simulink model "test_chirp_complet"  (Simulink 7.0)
settings: Solver=FixedStepDiscrete  StartTime=0.0  StopTime=50  FixedStep=Ts  RelTol=1e-3

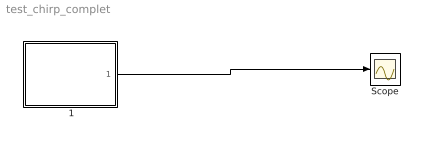
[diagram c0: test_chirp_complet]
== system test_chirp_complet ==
  " 1" : Subsystem  mask{n=2, Fbeg=[60; 90;75], Ffin=[70;100;85], amp=0.1, T0=15, T1=18, Tb=3, T2=3}
      mask prompts: n "level"; Fbeg "Initial frequency sequence (vector Fbeg) [Hz]"; Ffin "Final frequency sequence (vector Ffin) [Hz]"; amp "Amplitude (Amp)"; T0 "Instant of the initial frequency sequence injection 'T0'"; T1 "instant to run a chirp 'T1'"; Tb "Transition time between  Fbeg and Ffin ('Tb') "slope=(Ffin-Fbeg)/Tb""; T2 "Time duration of the final frequency sequence Ffin 'T2'"
  Scope : Scope
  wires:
  " 1"/1(Out2) -> Scope/1

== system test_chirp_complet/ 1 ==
  Constant : Constant  Value=n  OutDataType=sfix(16)  OutScaling=2^0
  Multiport Switch : MultiPortSwitch  Inputs=3  OutDataType=sfix(16)  OutScaling=2^0
  Subsystem : Subsystem
  Subsystem1 : Subsystem
  Subsystem2 : Subsystem
  Out2 : Outport
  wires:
  Constant/1 -> Multiport Switch/1
  Subsystem2/1(Out1) -> Multiport Switch/2
  Subsystem1/1(Out1) -> Multiport Switch/3
  Subsystem/1(Out1) -> Multiport Switch/4
  Multiport Switch/1 -> Out2/1

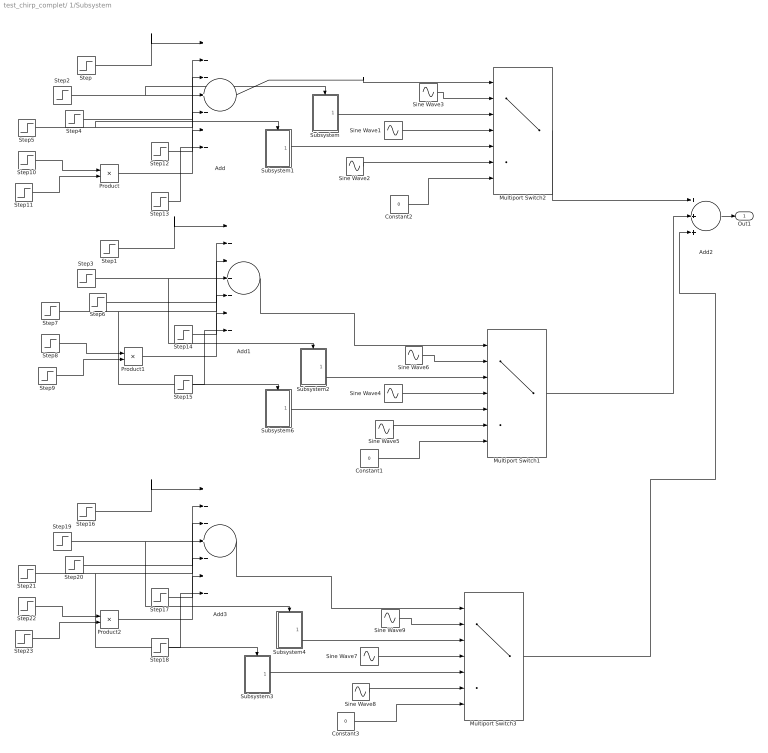
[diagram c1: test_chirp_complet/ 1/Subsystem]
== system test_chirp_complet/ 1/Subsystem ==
  Add : Sum  Inputs=+++++++  OutDataType=sfix(16)  OutScaling=2^-10
  Add1 : Sum  Inputs=+++++++  OutDataType=sfix(16)  OutScaling=2^-10
  Add2 : Sum  Inputs=+++  OutDataType=sfix(16)  OutScaling=2^-10
  Add3 : Sum  Inputs=+++++++  OutDataType=sfix(16)  OutScaling=2^-10
  Constant1 : Constant  Value=0  OutDataType=sfix(16)  OutScaling=2^0
  Constant2 : Constant  Value=0  OutDataType=sfix(16)  OutScaling=2^0
  Constant3 : Constant  Value=0  OutDataType=sfix(16)  OutScaling=2^0
  Multiport Switch1 : MultiPortSwitch  Inputs=6  OutDataType=sfix(16)  OutScaling=2^0
  Multiport Switch2 : MultiPortSwitch  Inputs=6  OutDataType=sfix(16)  OutScaling=2^0
  Multiport Switch3 : MultiPortSwitch  Inputs=6  OutDataType=sfix(16)  OutScaling=2^0
  Product : Product  OutDataType=sfix(16)  OutScaling=2^0
  Product1 : Product  OutDataType=sfix(16)  OutScaling=2^0
  Product2 : Product  OutDataType=sfix(16)  OutScaling=2^0
  Sine Wave1 : Sin  Amplitude=amp  Frequency=Ffin(1)*2*pi  SampleTime=0
  Sine Wave2 : Sin  Amplitude=amp  Frequency=Fbeg(1)*2*pi  SampleTime=0
  Sine Wave3 : Sin  Amplitude=amp  Frequency=Fbeg(1)*2*pi  SampleTime=0
  Sine Wave4 : Sin  Amplitude=amp  Frequency=Ffin(2)*2*pi  SampleTime=0
  Sine Wave5 : Sin  Amplitude=amp  Frequency=Fbeg(2)*2*pi  SampleTime=0
  Sine Wave6 : Sin  Amplitude=amp  Frequency=Fbeg(2)*2*pi  SampleTime=0
  Sine Wave7 : Sin  Amplitude=amp  Frequency=Ffin(3)*2*pi  SampleTime=0
  Sine Wave8 : Sin  Amplitude=amp  Frequency=Fbeg(3)*2*pi  SampleTime=0
  Sine Wave9 : Sin  Amplitude=amp  Frequency=Fbeg(3)*2*pi  SampleTime=0
  Step : Step  Time=T0  SampleTime=0
  Step1 : Step  Time=T0  SampleTime=0
  Step10 : Step  Time=0  After=4  SampleTime=0
  Step11 : Step  Time=T0  Before=1  After=0  SampleTime=0
  Step12 : Step  Time=Tb+T1+T2+Tb  SampleTime=0
  Step13 : Step  Time=Tb+T1+T2+Tb+T2  SampleTime=0
  Step14 : Step  Time=Tb+T1+T2+Tb  SampleTime=0
  Step15 : Step  Time=Tb+T1+T2+Tb+T2  SampleTime=0
  Step16 : Step  Time=T0  SampleTime=0
  Step17 : Step  Time=Tb+T1+T2+Tb  SampleTime=0
  Step18 : Step  Time=Tb+T1+T2+Tb+T2  SampleTime=0
  Step19 : Step  Time=T1  SampleTime=0
  Step2 : Step  Time=T1  SampleTime=0
  Step20 : Step  Time=Tb+T1  SampleTime=0
  Step21 : Step  Time=Tb+T1+T2  SampleTime=0
  Step22 : Step  Time=0  After=4  SampleTime=0
  Step23 : Step  Time=T0  Before=1  After=0  SampleTime=0
  Step3 : Step  Time=T1  SampleTime=0
  Step4 : Step  Time=Tb+T1  SampleTime=0
  Step5 : Step  Time=Tb+T1+T2  SampleTime=0
  Step6 : Step  Time=Tb+T1  SampleTime=0
  Step7 : Step  Time=Tb+T1+T2  SampleTime=0
  Step8 : Step  Time=0  After=4  SampleTime=0
  Step9 : Step  Time=T0  Before=1  After=0  SampleTime=0
  Subsystem : Subsystem
  Subsystem1 : Subsystem
  Subsystem2 : Subsystem
  Subsystem3 : Subsystem
  Subsystem4 : Subsystem
  Subsystem6 : Subsystem
  Out1 : Outport
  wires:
  Add2/1 -> Out1/1
  Subsystem/1(Out1) -> Multiport Switch2/3
  Sine Wave3/1 -> Multiport Switch2/2
  Sine Wave1/1 -> Multiport Switch2/4
  Subsystem1/1(Out1) -> Multiport Switch2/5
  Sine Wave2/1 -> Multiport Switch2/6
  Constant2/1 -> Multiport Switch2/7
  Step/1 -> Add/1
  Step2/1 -> Add/2, Subsystem/Enable
  Step4/1 -> Add/3
  Step5/1 -> Add/4, Subsystem1/Enable
  Step10/1 -> Product/1
  Step11/1 -> Product/2
  Add/1 -> Multiport Switch2/1
  Step12/1 -> Add/5
  Product/1 -> Add/6
  Multiport Switch2/1 -> Add2/1
  Step13/1 -> Add/7
  Subsystem2/1(Out1) -> Multiport Switch1/3
  Sine Wave6/1 -> Multiport Switch1/2
  Sine Wave4/1 -> Multiport Switch1/4
  Subsystem6/1(Out1) -> Multiport Switch1/5
  Sine Wave5/1 -> Multiport Switch1/6
  Constant1/1 -> Multiport Switch1/7
  Step1/1 -> Add1/1
  Step3/1 -> Add1/2, Subsystem2/Enable
  Step6/1 -> Add1/3
  Step7/1 -> Add1/4, Subsystem6/Enable
  Step8/1 -> Product1/1
  Step9/1 -> Product1/2
  Add1/1 -> Multiport Switch1/1
  Step14/1 -> Add1/5
  Product1/1 -> Add1/6
  Multiport Switch1/1 -> Add2/2
  Step15/1 -> Add1/7
  Subsystem4/1(Out1) -> Multiport Switch3/3
  Sine Wave9/1 -> Multiport Switch3/2
  Sine Wave7/1 -> Multiport Switch3/4
  Subsystem3/1(Out1) -> Multiport Switch3/5
  Sine Wave8/1 -> Multiport Switch3/6
  Constant3/1 -> Multiport Switch3/7
  Step16/1 -> Add3/1
  Step19/1 -> Add3/2, Subsystem4/Enable
  Step20/1 -> Add3/3
  Step21/1 -> Add3/4, Subsystem3/Enable
  Step22/1 -> Product2/1
  Step23/1 -> Product2/2
  Add3/1 -> Multiport Switch3/1
  Step17/1 -> Add3/5
  Product2/1 -> Add3/6
  Multiport Switch3/1 -> Add2/3
  Step18/1 -> Add3/7

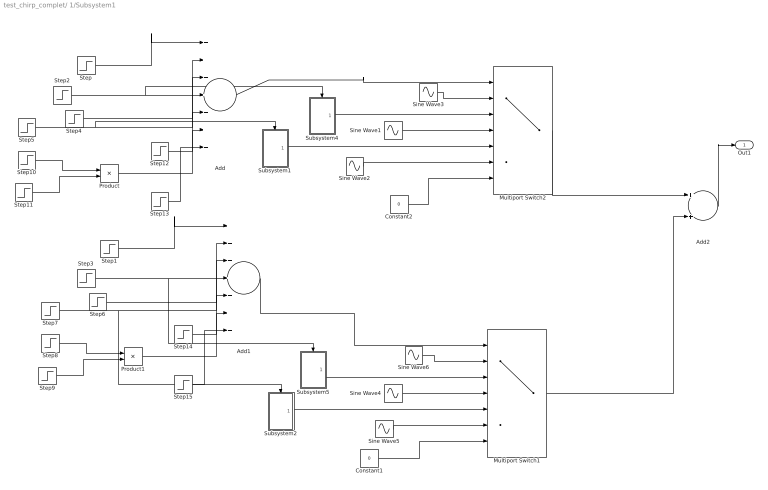
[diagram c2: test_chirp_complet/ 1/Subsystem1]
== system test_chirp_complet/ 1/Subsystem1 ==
  Add : Sum  Inputs=+++++++  OutDataType=sfix(16)  OutScaling=2^-10
  Add1 : Sum  Inputs=+++++++  OutDataType=sfix(16)  OutScaling=2^-10
  Add2 : Sum  OutDataType=sfix(16)  OutScaling=2^-10
  Constant1 : Constant  Value=0  OutDataType=sfix(16)  OutScaling=2^0
  Constant2 : Constant  Value=0  OutDataType=sfix(16)  OutScaling=2^0
  Multiport Switch1 : MultiPortSwitch  Inputs=6  OutDataType=sfix(16)  OutScaling=2^0
  Multiport Switch2 : MultiPortSwitch  Inputs=6  OutDataType=sfix(16)  OutScaling=2^0
  Product : Product  OutDataType=sfix(16)  OutScaling=2^0
  Product1 : Product  OutDataType=sfix(16)  OutScaling=2^0
  Sine Wave1 : Sin  Amplitude=amp  Frequency=Ffin(1)*2*pi  SampleTime=0
  Sine Wave2 : Sin  Amplitude=amp  Frequency=Fbeg(1)*2*pi  SampleTime=0
  Sine Wave3 : Sin  Amplitude=amp  Frequency=Fbeg(1)*2*pi  SampleTime=0
  Sine Wave4 : Sin  Amplitude=amp  Frequency=Ffin(2)*2*pi  SampleTime=0
  Sine Wave5 : Sin  Amplitude=amp  Frequency=Fbeg(2)*2*pi  SampleTime=0
  Sine Wave6 : Sin  Amplitude=amp  Frequency=Fbeg(2)*2*pi  SampleTime=0
  Step : Step  Time=T0  SampleTime=0
  Step1 : Step  Time=T0  SampleTime=0
  Step10 : Step  Time=0  After=4  SampleTime=0
  Step11 : Step  Time=T0  Before=1  After=0  SampleTime=0
  Step12 : Step  Time=Tb+T1+T2+Tb  SampleTime=0
  Step13 : Step  Time=Tb+T1+T2+Tb+T2  SampleTime=0
  Step14 : Step  Time=Tb+T1+T2+Tb  SampleTime=0
  Step15 : Step  Time=Tb+T1+T2+Tb+T2  SampleTime=0
  Step2 : Step  Time=T1  SampleTime=0
  Step3 : Step  Time=T1  SampleTime=0
  Step4 : Step  Time=Tb+T1  SampleTime=0
  Step5 : Step  Time=Tb+T1+T2  SampleTime=0
  Step6 : Step  Time=Tb+T1  SampleTime=0
  Step7 : Step  Time=Tb+T1+T2  SampleTime=0
  Step8 : Step  Time=0  After=4  SampleTime=0
  Step9 : Step  Time=T0  Before=1  After=0  SampleTime=0
  Subsystem1 : Subsystem
  Subsystem2 : Subsystem
  Subsystem4 : Subsystem
  Subsystem5 : Subsystem
  Out1 : Outport
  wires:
  Add2/1 -> Out1/1
  Subsystem4/1(Out1) -> Multiport Switch2/3
  Sine Wave3/1 -> Multiport Switch2/2
  Sine Wave1/1 -> Multiport Switch2/4
  Subsystem1/1(Out1) -> Multiport Switch2/5
  Sine Wave2/1 -> Multiport Switch2/6
  Constant2/1 -> Multiport Switch2/7
  Step/1 -> Add/1
  Step2/1 -> Add/2, Subsystem4/Enable
  Step4/1 -> Add/3
  Step5/1 -> Add/4, Subsystem1/Enable
  Step10/1 -> Product/1
  Step11/1 -> Product/2
  Add/1 -> Multiport Switch2/1
  Step12/1 -> Add/5
  Product/1 -> Add/6
  Multiport Switch2/1 -> Add2/1
  Step13/1 -> Add/7
  Subsystem5/1(Out1) -> Multiport Switch1/3
  Sine Wave6/1 -> Multiport Switch1/2
  Sine Wave4/1 -> Multiport Switch1/4
  Subsystem2/1(Out1) -> Multiport Switch1/5
  Sine Wave5/1 -> Multiport Switch1/6
  Constant1/1 -> Multiport Switch1/7
  Step1/1 -> Add1/1
  Step3/1 -> Add1/2, Subsystem5/Enable
  Step6/1 -> Add1/3
  Step7/1 -> Add1/4, Subsystem2/Enable
  Step8/1 -> Product1/1
  Step9/1 -> Product1/2
  Add1/1 -> Multiport Switch1/1
  Step14/1 -> Add1/5
  Product1/1 -> Add1/6
  Multiport Switch1/1 -> Add2/2
  Step15/1 -> Add1/7

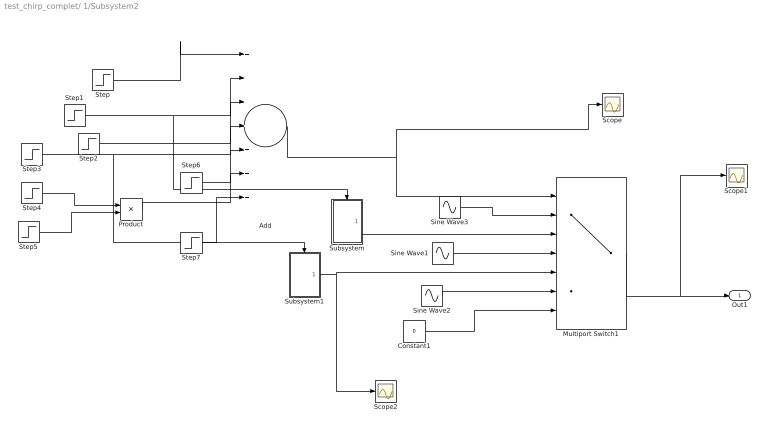
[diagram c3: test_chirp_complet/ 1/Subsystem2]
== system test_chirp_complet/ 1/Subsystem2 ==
  Add : Sum  Inputs=+++++++  OutDataType=sfix(16)  OutScaling=2^-10
  Constant1 : Constant  Value=0  OutDataType=sfix(16)  OutScaling=2^0
  Multiport Switch1 : MultiPortSwitch  Inputs=6  OutDataType=sfix(16)  OutScaling=2^0
  Product : Product  OutDataType=sfix(16)  OutScaling=2^0
  Scope : Scope
  Scope1 : Scope
  Scope2 : Scope
  Sine Wave1 : Sin  Amplitude=amp  Frequency=Ffin(1)*2*pi  SampleTime=0
  Sine Wave2 : Sin  Amplitude=amp  Frequency=Fbeg(1)*2*pi  SampleTime=0
  Sine Wave3 : Sin  Amplitude=amp  Frequency=Fbeg(1)*2*pi  SampleTime=0
  Step : Step  Time=T0  SampleTime=0
  Step1 : Step  Time=T1  SampleTime=0
  Step2 : Step  Time=Tb+T1  SampleTime=0
  Step3 : Step  Time=Tb+T1+T2  SampleTime=0
  Step4 : Step  Time=0  After=4  SampleTime=0
  Step5 : Step  Time=T0  Before=1  After=0  SampleTime=0
  Step6 : Step  Time=Tb+T1+T2+Tb  SampleTime=0
  Step7 : Step  Time=Tb+T1+T2+Tb+T2  SampleTime=0
  Subsystem : Subsystem
  Subsystem1 : Subsystem
  Out1 : Outport
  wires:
  Subsystem/1(Out1) -> Multiport Switch1/3
  Sine Wave3/1 -> Multiport Switch1/2
  Sine Wave1/1 -> Multiport Switch1/4
  Subsystem1/1(Out1) -> Multiport Switch1/5, Scope2/1
  Sine Wave2/1 -> Multiport Switch1/6
  Constant1/1 -> Multiport Switch1/7
  Step/1 -> Add/1
  Step1/1 -> Add/2, Subsystem/Enable
  Step2/1 -> Add/3
  Step3/1 -> Add/4, Subsystem1/Enable
  Step4/1 -> Product/1
  Step5/1 -> Product/2
  Add/1 -> Multiport Switch1/1, Scope/1
  Step6/1 -> Add/5
  Product/1 -> Add/6
  Multiport Switch1/1 -> Out1/1, Scope1/1
  Step7/1 -> Add/7

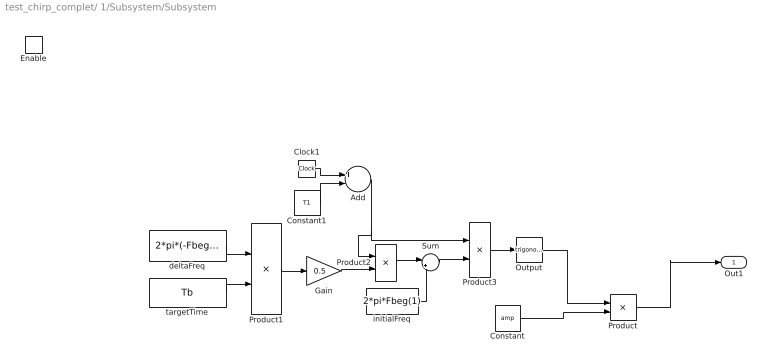
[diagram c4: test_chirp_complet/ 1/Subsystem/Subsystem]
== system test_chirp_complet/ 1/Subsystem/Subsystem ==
  Enable : EnablePort
  Add : Sum  Inputs=+-  OutDataType=sfix(16)  OutScaling=2^-10
  Clock1 : Clock
  Constant : Constant  Value=amp  OutDataType=sfix(16)  OutScaling=2^0
  Constant1 : Constant  Value=T1  OutDataType=sfix(16)  OutScaling=2^0
  Gain : Gain  Gain=0.5  ParameterDataType=sfix(16)  ParameterScaling=2^0  OutDataType=sfix(16)  OutScaling=2^0
  Output : Trigonometry
  Product : Product  OutDataType=sfix(16)  OutScaling=2^0
  Product1 : Product  Inputs=*/  OutDataType=sfix(16)  OutScaling=2^0
  Product2 : Product  OutDataType=sfix(16)  OutScaling=2^0
  Product3 : Product  OutDataType=sfix(16)  OutScaling=2^0
  Sum : Sum  Inputs=|++  OutDataType=sfix(16)  OutScaling=2^0
  deltaFreq : Constant  Value=2*pi*(-Fbeg(1)+Ffin(1))  OutDataType=sfix(16)  OutScaling=2^0
  initialFreq : Constant  Value=2*pi*Fbeg(1)  OutDataType=sfix(16)  OutScaling=2^0
  targetTime : Constant  Value=Tb  OutDataType=sfix(16)  OutScaling=2^0
  Out1 : Outport
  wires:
  Constant/1 -> Product/2
  Output/1 -> Product/1
  Product/1 -> Out1/1
  Product3/1 -> Output/1
  Sum/1 -> Product3/2
  initialFreq/1 -> Sum/2
  Product2/1 -> Sum/1
  Gain/1 -> Product2/2
  Product1/1 -> Gain/1
  targetTime/1 -> Product1/2
  deltaFreq/1 -> Product1/1
  Clock1/1 -> Add/1
  Constant1/1 -> Add/2
  Add/1 -> Product2/1, Product3/1

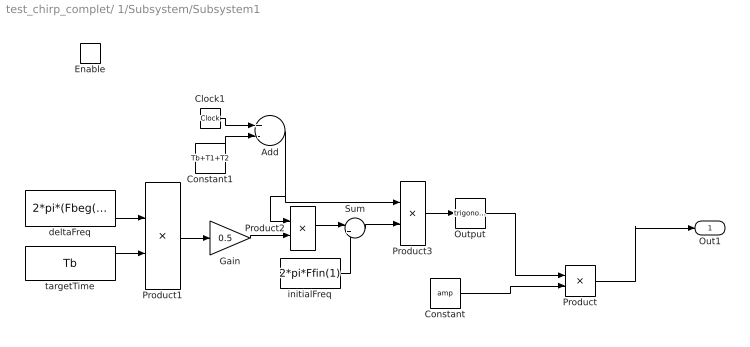
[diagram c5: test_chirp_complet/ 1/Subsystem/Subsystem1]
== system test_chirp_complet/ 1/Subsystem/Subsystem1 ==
  Enable : EnablePort
  Add : Sum  Inputs=+-  OutDataType=sfix(16)  OutScaling=2^-10
  Clock1 : Clock
  Constant : Constant  Value=amp  OutDataType=sfix(16)  OutScaling=2^0
  Constant1 : Constant  Value=Tb+T1+T2  OutDataType=sfix(16)  OutScaling=2^0
  Gain : Gain  Gain=0.5  ParameterDataType=sfix(16)  ParameterScaling=2^0  OutDataType=sfix(16)  OutScaling=2^0
  Output : Trigonometry
  Product : Product  OutDataType=sfix(16)  OutScaling=2^0
  Product1 : Product  Inputs=*/  OutDataType=sfix(16)  OutScaling=2^0
  Product2 : Product  OutDataType=sfix(16)  OutScaling=2^0
  Product3 : Product  OutDataType=sfix(16)  OutScaling=2^0
  Sum : Sum  Inputs=|++  OutDataType=sfix(16)  OutScaling=2^0
  deltaFreq : Constant  Value=2*pi*(Fbeg(1)-Ffin(1))  OutDataType=sfix(16)  OutScaling=2^0
  initialFreq : Constant  Value=2*pi*Ffin(1)  OutDataType=sfix(16)  OutScaling=2^0
  targetTime : Constant  Value=Tb  OutDataType=sfix(16)  OutScaling=2^0
  Out1 : Outport
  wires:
  Add/1 -> Product3/1, Product2/1
  Constant1/1 -> Add/2
  Clock1/1 -> Add/1
  deltaFreq/1 -> Product1/1
  targetTime/1 -> Product1/2
  Product1/1 -> Gain/1
  Gain/1 -> Product2/2
  Product2/1 -> Sum/1
  initialFreq/1 -> Sum/2
  Sum/1 -> Product3/2
  Product3/1 -> Output/1
  Product/1 -> Out1/1
  Output/1 -> Product/1
  Constant/1 -> Product/2

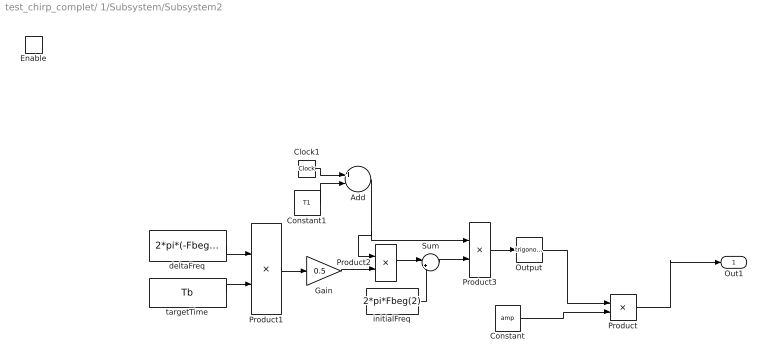
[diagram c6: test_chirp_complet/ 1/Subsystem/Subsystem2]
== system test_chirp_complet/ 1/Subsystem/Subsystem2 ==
  Enable : EnablePort
  Add : Sum  Inputs=+-  OutDataType=sfix(16)  OutScaling=2^-10
  Clock1 : Clock
  Constant : Constant  Value=amp  OutDataType=sfix(16)  OutScaling=2^0
  Constant1 : Constant  Value=T1  OutDataType=sfix(16)  OutScaling=2^0
  Gain : Gain  Gain=0.5  ParameterDataType=sfix(16)  ParameterScaling=2^0  OutDataType=sfix(16)  OutScaling=2^0
  Output : Trigonometry
  Product : Product  OutDataType=sfix(16)  OutScaling=2^0
  Product1 : Product  Inputs=*/  OutDataType=sfix(16)  OutScaling=2^0
  Product2 : Product  OutDataType=sfix(16)  OutScaling=2^0
  Product3 : Product  OutDataType=sfix(16)  OutScaling=2^0
  Sum : Sum  Inputs=|++  OutDataType=sfix(16)  OutScaling=2^0
  deltaFreq : Constant  Value=2*pi*(-Fbeg(2)+Ffin(2))  OutDataType=sfix(16)  OutScaling=2^0
  initialFreq : Constant  Value=2*pi*Fbeg(2)  OutDataType=sfix(16)  OutScaling=2^0
  targetTime : Constant  Value=Tb  OutDataType=sfix(16)  OutScaling=2^0
  Out1 : Outport
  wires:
  Add/1 -> Product3/1, Product2/1
  Constant1/1 -> Add/2
  Clock1/1 -> Add/1
  deltaFreq/1 -> Product1/1
  targetTime/1 -> Product1/2
  Product1/1 -> Gain/1
  Gain/1 -> Product2/2
  Product2/1 -> Sum/1
  initialFreq/1 -> Sum/2
  Sum/1 -> Product3/2
  Product3/1 -> Output/1
  Product/1 -> Out1/1
  Output/1 -> Product/1
  Constant/1 -> Product/2

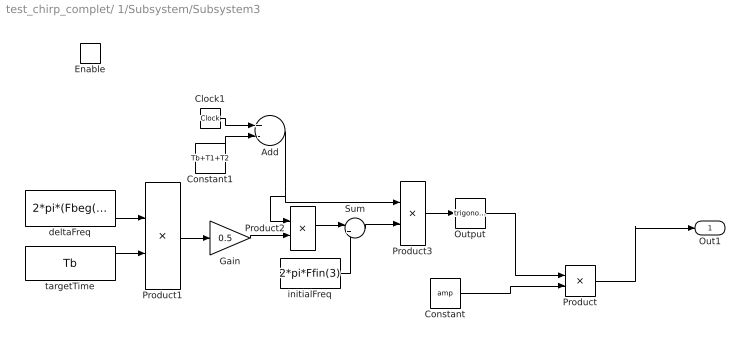
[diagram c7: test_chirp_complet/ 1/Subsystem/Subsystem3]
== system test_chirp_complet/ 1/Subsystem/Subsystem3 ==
  Enable : EnablePort
  Add : Sum  Inputs=+-  OutDataType=sfix(16)  OutScaling=2^-10
  Clock1 : Clock
  Constant : Constant  Value=amp  OutDataType=sfix(16)  OutScaling=2^0
  Constant1 : Constant  Value=Tb+T1+T2  OutDataType=sfix(16)  OutScaling=2^0
  Gain : Gain  Gain=0.5  ParameterDataType=sfix(16)  ParameterScaling=2^0  OutDataType=sfix(16)  OutScaling=2^0
  Output : Trigonometry
  Product : Product  OutDataType=sfix(16)  OutScaling=2^0
  Product1 : Product  Inputs=*/  OutDataType=sfix(16)  OutScaling=2^0
  Product2 : Product  OutDataType=sfix(16)  OutScaling=2^0
  Product3 : Product  OutDataType=sfix(16)  OutScaling=2^0
  Sum : Sum  Inputs=|++  OutDataType=sfix(16)  OutScaling=2^0
  deltaFreq : Constant  Value=2*pi*(Fbeg(3)-Ffin(3))  OutDataType=sfix(16)  OutScaling=2^0
  initialFreq : Constant  Value=2*pi*Ffin(3)  OutDataType=sfix(16)  OutScaling=2^0
  targetTime : Constant  Value=Tb  OutDataType=sfix(16)  OutScaling=2^0
  Out1 : Outport
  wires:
  Add/1 -> Product3/1, Product2/1
  Constant1/1 -> Add/2
  Clock1/1 -> Add/1
  deltaFreq/1 -> Product1/1
  targetTime/1 -> Product1/2
  Product1/1 -> Gain/1
  Gain/1 -> Product2/2
  Product2/1 -> Sum/1
  initialFreq/1 -> Sum/2
  Sum/1 -> Product3/2
  Product3/1 -> Output/1
  Product/1 -> Out1/1
  Output/1 -> Product/1
  Constant/1 -> Product/2

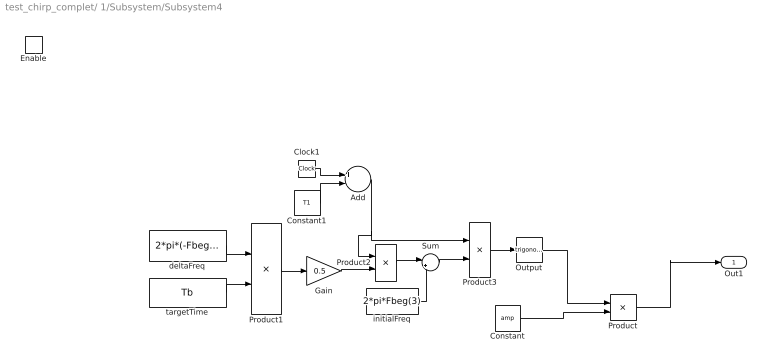
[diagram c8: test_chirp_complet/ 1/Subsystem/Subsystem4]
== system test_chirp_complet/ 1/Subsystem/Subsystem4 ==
  Enable : EnablePort
  Add : Sum  Inputs=+-  OutDataType=sfix(16)  OutScaling=2^-10
  Clock1 : Clock
  Constant : Constant  Value=amp  OutDataType=sfix(16)  OutScaling=2^0
  Constant1 : Constant  Value=T1  OutDataType=sfix(16)  OutScaling=2^0
  Gain : Gain  Gain=0.5  ParameterDataType=sfix(16)  ParameterScaling=2^0  OutDataType=sfix(16)  OutScaling=2^0
  Output : Trigonometry
  Product : Product  OutDataType=sfix(16)  OutScaling=2^0
  Product1 : Product  Inputs=*/  OutDataType=sfix(16)  OutScaling=2^0
  Product2 : Product  OutDataType=sfix(16)  OutScaling=2^0
  Product3 : Product  OutDataType=sfix(16)  OutScaling=2^0
  Sum : Sum  Inputs=|++  OutDataType=sfix(16)  OutScaling=2^0
  deltaFreq : Constant  Value=2*pi*(-Fbeg(3)+Ffin(3))  OutDataType=sfix(16)  OutScaling=2^0
  initialFreq : Constant  Value=2*pi*Fbeg(3)  OutDataType=sfix(16)  OutScaling=2^0
  targetTime : Constant  Value=Tb  OutDataType=sfix(16)  OutScaling=2^0
  Out1 : Outport
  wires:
  Constant/1 -> Product/2
  Output/1 -> Product/1
  Product/1 -> Out1/1
  Product3/1 -> Output/1
  Sum/1 -> Product3/2
  initialFreq/1 -> Sum/2
  Product2/1 -> Sum/1
  Gain/1 -> Product2/2
  Product1/1 -> Gain/1
  targetTime/1 -> Product1/2
  deltaFreq/1 -> Product1/1
  Clock1/1 -> Add/1
  Constant1/1 -> Add/2
  Add/1 -> Product2/1, Product3/1

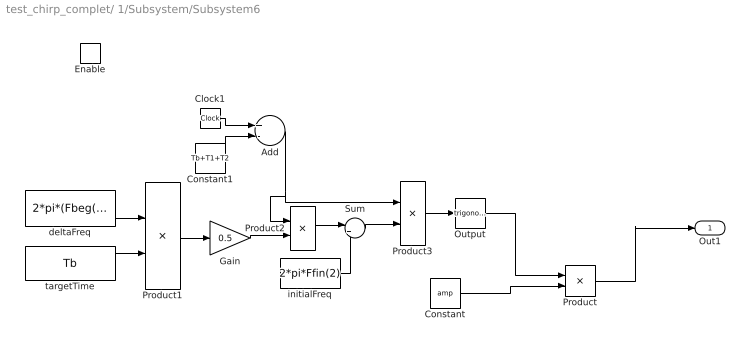
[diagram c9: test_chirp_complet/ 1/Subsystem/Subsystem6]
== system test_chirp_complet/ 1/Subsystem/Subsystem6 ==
  Enable : EnablePort
  Add : Sum  Inputs=+-  OutDataType=sfix(16)  OutScaling=2^-10
  Clock1 : Clock
  Constant : Constant  Value=amp  OutDataType=sfix(16)  OutScaling=2^0
  Constant1 : Constant  Value=Tb+T1+T2  OutDataType=sfix(16)  OutScaling=2^0
  Gain : Gain  Gain=0.5  ParameterDataType=sfix(16)  ParameterScaling=2^0  OutDataType=sfix(16)  OutScaling=2^0
  Output : Trigonometry
  Product : Product  OutDataType=sfix(16)  OutScaling=2^0
  Product1 : Product  Inputs=*/  OutDataType=sfix(16)  OutScaling=2^0
  Product2 : Product  OutDataType=sfix(16)  OutScaling=2^0
  Product3 : Product  OutDataType=sfix(16)  OutScaling=2^0
  Sum : Sum  Inputs=|++  OutDataType=sfix(16)  OutScaling=2^0
  deltaFreq : Constant  Value=2*pi*(Fbeg(2)-Ffin(2))  OutDataType=sfix(16)  OutScaling=2^0
  initialFreq : Constant  Value=2*pi*Ffin(2)  OutDataType=sfix(16)  OutScaling=2^0
  targetTime : Constant  Value=Tb  OutDataType=sfix(16)  OutScaling=2^0
  Out1 : Outport
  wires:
  Constant/1 -> Product/2
  Output/1 -> Product/1
  Product/1 -> Out1/1
  Product3/1 -> Output/1
  Sum/1 -> Product3/2
  initialFreq/1 -> Sum/2
  Product2/1 -> Sum/1
  Gain/1 -> Product2/2
  Product1/1 -> Gain/1
  targetTime/1 -> Product1/2
  deltaFreq/1 -> Product1/1
  Clock1/1 -> Add/1
  Constant1/1 -> Add/2
  Add/1 -> Product2/1, Product3/1

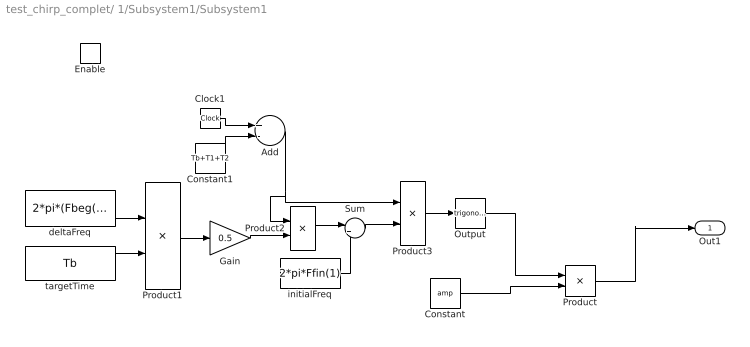
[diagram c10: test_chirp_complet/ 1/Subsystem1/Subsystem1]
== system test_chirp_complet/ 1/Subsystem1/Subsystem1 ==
  Enable : EnablePort
  Add : Sum  Inputs=+-  OutDataType=sfix(16)  OutScaling=2^-10
  Clock1 : Clock
  Constant : Constant  Value=amp  OutDataType=sfix(16)  OutScaling=2^0
  Constant1 : Constant  Value=Tb+T1+T2  OutDataType=sfix(16)  OutScaling=2^0
  Gain : Gain  Gain=0.5  ParameterDataType=sfix(16)  ParameterScaling=2^0  OutDataType=sfix(16)  OutScaling=2^0
  Output : Trigonometry
  Product : Product  OutDataType=sfix(16)  OutScaling=2^0
  Product1 : Product  Inputs=*/  OutDataType=sfix(16)  OutScaling=2^0
  Product2 : Product  OutDataType=sfix(16)  OutScaling=2^0
  Product3 : Product  OutDataType=sfix(16)  OutScaling=2^0
  Sum : Sum  Inputs=|++  OutDataType=sfix(16)  OutScaling=2^0
  deltaFreq : Constant  Value=2*pi*(Fbeg(1)-Ffin(1))  OutDataType=sfix(16)  OutScaling=2^0
  initialFreq : Constant  Value=2*pi*Ffin(1)  OutDataType=sfix(16)  OutScaling=2^0
  targetTime : Constant  Value=Tb  OutDataType=sfix(16)  OutScaling=2^0
  Out1 : Outport
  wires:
  Constant/1 -> Product/2
  Output/1 -> Product/1
  Product/1 -> Out1/1
  Product3/1 -> Output/1
  Sum/1 -> Product3/2
  initialFreq/1 -> Sum/2
  Product2/1 -> Sum/1
  Gain/1 -> Product2/2
  Product1/1 -> Gain/1
  targetTime/1 -> Product1/2
  deltaFreq/1 -> Product1/1
  Clock1/1 -> Add/1
  Constant1/1 -> Add/2
  Add/1 -> Product2/1, Product3/1

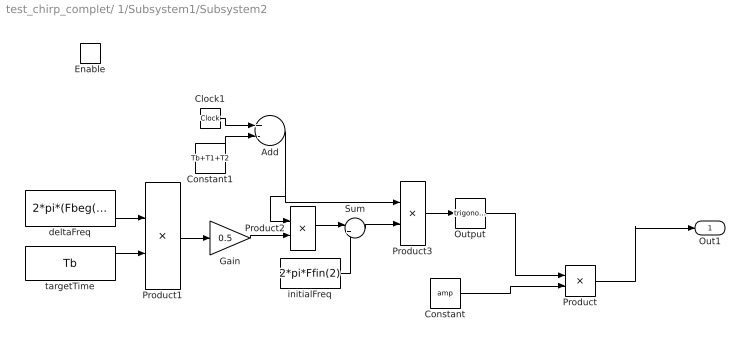
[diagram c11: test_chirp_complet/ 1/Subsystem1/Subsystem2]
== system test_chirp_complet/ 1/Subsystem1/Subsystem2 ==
  Enable : EnablePort
  Add : Sum  Inputs=+-  OutDataType=sfix(16)  OutScaling=2^-10
  Clock1 : Clock
  Constant : Constant  Value=amp  OutDataType=sfix(16)  OutScaling=2^0
  Constant1 : Constant  Value=Tb+T1+T2  OutDataType=sfix(16)  OutScaling=2^0
  Gain : Gain  Gain=0.5  ParameterDataType=sfix(16)  ParameterScaling=2^0  OutDataType=sfix(16)  OutScaling=2^0
  Output : Trigonometry
  Product : Product  OutDataType=sfix(16)  OutScaling=2^0
  Product1 : Product  Inputs=*/  OutDataType=sfix(16)  OutScaling=2^0
  Product2 : Product  OutDataType=sfix(16)  OutScaling=2^0
  Product3 : Product  OutDataType=sfix(16)  OutScaling=2^0
  Sum : Sum  Inputs=|++  OutDataType=sfix(16)  OutScaling=2^0
  deltaFreq : Constant  Value=2*pi*(Fbeg(2)-Ffin(2))  OutDataType=sfix(16)  OutScaling=2^0
  initialFreq : Constant  Value=2*pi*Ffin(2)  OutDataType=sfix(16)  OutScaling=2^0
  targetTime : Constant  Value=Tb  OutDataType=sfix(16)  OutScaling=2^0
  Out1 : Outport
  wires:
  Add/1 -> Product3/1, Product2/1
  Constant1/1 -> Add/2
  Clock1/1 -> Add/1
  deltaFreq/1 -> Product1/1
  targetTime/1 -> Product1/2
  Product1/1 -> Gain/1
  Gain/1 -> Product2/2
  Product2/1 -> Sum/1
  initialFreq/1 -> Sum/2
  Sum/1 -> Product3/2
  Product3/1 -> Output/1
  Product/1 -> Out1/1
  Output/1 -> Product/1
  Constant/1 -> Product/2

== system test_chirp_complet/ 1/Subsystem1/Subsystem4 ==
  Enable : EnablePort
  Add : Sum  Inputs=+-  OutDataType=sfix(16)  OutScaling=2^-10
  Clock1 : Clock
  Constant : Constant  Value=amp  OutDataType=sfix(16)  OutScaling=2^0
  Constant1 : Constant  Value=T1  OutDataType=sfix(16)  OutScaling=2^0
  Gain : Gain  Gain=0.5  ParameterDataType=sfix(16)  ParameterScaling=2^0  OutDataType=sfix(16)  OutScaling=2^0
  Output : Trigonometry
  Product : Product  OutDataType=sfix(16)  OutScaling=2^0
  Product1 : Product  Inputs=*/  OutDataType=sfix(16)  OutScaling=2^0
  Product2 : Product  OutDataType=sfix(16)  OutScaling=2^0
  Product3 : Product  OutDataType=sfix(16)  OutScaling=2^0
  Sum : Sum  Inputs=|++  OutDataType=sfix(16)  OutScaling=2^0
  deltaFreq : Constant  Value=2*pi*(-Fbeg(1)+Ffin(1))  OutDataType=sfix(16)  OutScaling=2^0
  initialFreq : Constant  Value=2*pi*Fbeg(1)  OutDataType=sfix(16)  OutScaling=2^0
  targetTime : Constant  Value=Tb  OutDataType=sfix(16)  OutScaling=2^0
  Out1 : Outport
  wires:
  Constant/1 -> Product/2
  Output/1 -> Product/1
  Product/1 -> Out1/1
  Product3/1 -> Output/1
  Sum/1 -> Product3/2
  initialFreq/1 -> Sum/2
  Product2/1 -> Sum/1
  Gain/1 -> Product2/2
  Product1/1 -> Gain/1
  targetTime/1 -> Product1/2
  deltaFreq/1 -> Product1/1
  Clock1/1 -> Add/1
  Constant1/1 -> Add/2
  Add/1 -> Product2/1, Product3/1

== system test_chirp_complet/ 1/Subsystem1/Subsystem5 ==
  Enable : EnablePort
  Add : Sum  Inputs=+-  OutDataType=sfix(16)  OutScaling=2^-10
  Clock1 : Clock
  Constant : Constant  Value=amp  OutDataType=sfix(16)  OutScaling=2^0
  Constant1 : Constant  Value=T1  OutDataType=sfix(16)  OutScaling=2^0
  Gain : Gain  Gain=0.5  ParameterDataType=sfix(16)  ParameterScaling=2^0  OutDataType=sfix(16)  OutScaling=2^0
  Output : Trigonometry
  Product : Product  OutDataType=sfix(16)  OutScaling=2^0
  Product1 : Product  Inputs=*/  OutDataType=sfix(16)  OutScaling=2^0
  Product2 : Product  OutDataType=sfix(16)  OutScaling=2^0
  Product3 : Product  OutDataType=sfix(16)  OutScaling=2^0
  Sum : Sum  Inputs=|++  OutDataType=sfix(16)  OutScaling=2^0
  deltaFreq : Constant  Value=2*pi*(-Fbeg(2)+Ffin(2))  OutDataType=sfix(16)  OutScaling=2^0
  initialFreq : Constant  Value=2*pi*Fbeg(2)  OutDataType=sfix(16)  OutScaling=2^0
  targetTime : Constant  Value=Tb  OutDataType=sfix(16)  OutScaling=2^0
  Out1 : Outport
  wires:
  Add/1 -> Product3/1, Product2/1
  Constant1/1 -> Add/2
  Clock1/1 -> Add/1
  deltaFreq/1 -> Product1/1
  targetTime/1 -> Product1/2
  Product1/1 -> Gain/1
  Gain/1 -> Product2/2
  Product2/1 -> Sum/1
  initialFreq/1 -> Sum/2
  Sum/1 -> Product3/2
  Product3/1 -> Output/1
  Product/1 -> Out1/1
  Output/1 -> Product/1
  Constant/1 -> Product/2

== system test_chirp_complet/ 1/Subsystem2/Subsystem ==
  Enable : EnablePort
  Add : Sum  Inputs=+-  OutDataType=sfix(16)  OutScaling=2^-10
  Clock1 : Clock
  Constant : Constant  Value=amp  OutDataType=sfix(16)  OutScaling=2^0
  Constant1 : Constant  Value=T1  OutDataType=sfix(16)  OutScaling=2^0
  Gain : Gain  Gain=0.5  ParameterDataType=sfix(16)  ParameterScaling=2^0  OutDataType=sfix(16)  OutScaling=2^0
  Output : Trigonometry
  Product : Product  OutDataType=sfix(16)  OutScaling=2^0
  Product1 : Product  Inputs=*/  OutDataType=sfix(16)  OutScaling=2^0
  Product2 : Product  OutDataType=sfix(16)  OutScaling=2^0
  Product3 : Product  OutDataType=sfix(16)  OutScaling=2^0
  Sum : Sum  Inputs=|++  OutDataType=sfix(16)  OutScaling=2^0
  deltaFreq : Constant  Value=2*pi*(-Fbeg(1)+Ffin(1))  OutDataType=sfix(16)  OutScaling=2^0
  initialFreq : Constant  Value=2*pi*Fbeg(1)  OutDataType=sfix(16)  OutScaling=2^0
  targetTime : Constant  Value=Tb  OutDataType=sfix(16)  OutScaling=2^0
  Out1 : Outport
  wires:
  Constant/1 -> Product/2
  Output/1 -> Product/1
  Product/1 -> Out1/1
  Product3/1 -> Output/1
  Sum/1 -> Product3/2
  initialFreq/1 -> Sum/2
  Product2/1 -> Sum/1
  Gain/1 -> Product2/2
  Product1/1 -> Gain/1
  targetTime/1 -> Product1/2
  deltaFreq/1 -> Product1/1
  Clock1/1 -> Add/1
  Constant1/1 -> Add/2
  Add/1 -> Product2/1, Product3/1

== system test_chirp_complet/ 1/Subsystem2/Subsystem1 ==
  Enable : EnablePort
  Add : Sum  Inputs=+-  OutDataType=sfix(16)  OutScaling=2^-10
  Clock1 : Clock
  Constant : Constant  Value=amp  OutDataType=sfix(16)  OutScaling=2^0
  Constant1 : Constant  Value=Tb+T1+T2  OutDataType=sfix(16)  OutScaling=2^0
  Gain : Gain  Gain=0.5  ParameterDataType=sfix(16)  ParameterScaling=2^0  OutDataType=sfix(16)  OutScaling=2^0
  Output : Trigonometry
  Product : Product  OutDataType=sfix(16)  OutScaling=2^0
  Product1 : Product  Inputs=*/  OutDataType=sfix(16)  OutScaling=2^0
  Product2 : Product  OutDataType=sfix(16)  OutScaling=2^0
  Product3 : Product  OutDataType=sfix(16)  OutScaling=2^0
  Sum : Sum  Inputs=|++  OutDataType=sfix(16)  OutScaling=2^0
  deltaFreq : Constant  Value=2*pi*(Fbeg(1)-Ffin(1))  OutDataType=sfix(16)  OutScaling=2^0
  initialFreq : Constant  Value=2*pi*Ffin(1)  OutDataType=sfix(16)  OutScaling=2^0
  targetTime : Constant  Value=Tb  OutDataType=sfix(16)  OutScaling=2^0
  Out1 : Outport
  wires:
  Constant/1 -> Product/2
  Output/1 -> Product/1
  Product/1 -> Out1/1
  Product3/1 -> Output/1
  Sum/1 -> Product3/2
  initialFreq/1 -> Sum/2
  Product2/1 -> Sum/1
  Gain/1 -> Product2/2
  Product1/1 -> Gain/1
  targetTime/1 -> Product1/2
  deltaFreq/1 -> Product1/1
  Clock1/1 -> Add/1
  Constant1/1 -> Add/2
  Add/1 -> Product2/1, Product3/1
